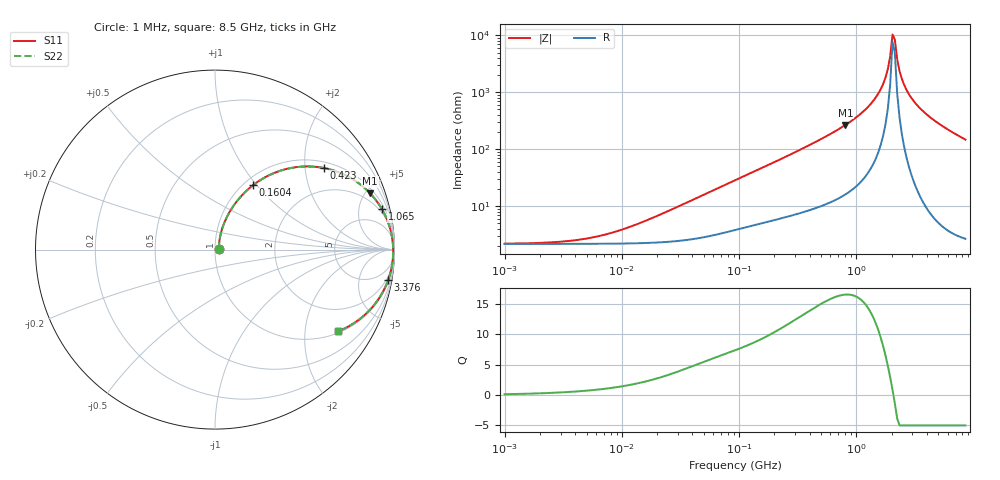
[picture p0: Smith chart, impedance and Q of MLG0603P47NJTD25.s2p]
! S-Parameter Data Generated by TDK Corporation
! Copyright(C) 2025 TDK Corporation.
! All Rights Reserved.
! TDK P/N: MLG0603P47NJTD25 (SMD / SMT Inductor (Coil))
! Property: L=47nH at 300MHz
! Size(LxWxT): 0.6x0.3x0.3mm
! Model Type: s2p (Touchstone File Format Version 1.0)
! Frequency: DC=Yes Start=1MHz Stop=8500MHz 198points Log-sweep
! Model Generated on Feb. 6, 2025
! Terms and conditions regarding TDK Simulation Models:
! 1)This simulation model is being provided solely for informational
!  purposes. Please refer to the specifications of the products in
!  terms of detailed characteristics of such products.
! 2)In no event shall TDK Corporation of any of its subsidiaries be
!  liable for any loss or damage arising, directly or indirectly,
!  from any information contained in this simulation model, including,
!  but not limited to loss or damages arising from any inaccuracies,
!  omissions or errors in connection with such information.
! 3)Any and all copyrights on this simulation model are owned by
!  TDK Corporation.  Duplication or redistribution of this simulation
!  model without prior written permission from TDK Corporation
!  is prohibited.
! 4)This simulation model is subject to any modification or change
!  without any prior notice.
! 5)Neither TDK Corporation nor any of its subsidiaries shall make any
!  warranty, express or implied, including but not limited to the
!  correctness, implied warranties of merchantability and fitness for
!  a particular purpose with respect to this simulation models.
! 6)The use of this simulation model shall be deemed to have consented
!  to the terms and conditions hereof.
! Port Assignments:
!  1 ---@@@--- 2
! Applicable Conditions:
!  Temperature = 25 degC
!  DC Bias Current = 0 A
!  Small Signal Operation
# Hz S MA R 50
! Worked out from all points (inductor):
!   197 points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, 1 MHz to 8.5 GHz, reference 50 ohm
!   read as one part in series: L = 50.5 nH near 22.04 MHz
!   highest Q = 16.6 at 807.2 MHz (marker M1), where L = 52.8 nH
!   self-resonance near 2.032 GHz
!   S11 on the Smith chart (normalised r, x): 1 MHz: 1.04, +0.01; 160.4 MHz: 1.10, +0.96; 423 MHz: 1.18, +2.52; 1.065 GHz: 1.51, +8.10; 3.376 GHz: 1, -11; 8.5 GHz: 1.05, -2.96
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1000000  0.02157 8.2  0.9787 -0.2  0.9787 -0.2  0.02157 8.2
4587603  0.02576 33.0  0.9785 -0.8  0.9785 -0.8  0.02576 33.0
9168677  0.03586 51.3  0.978 -1.6  0.978 -1.6  0.03586 51.3
2.10461e7  0.06914 67.1  0.9752 -3.7  0.9752 -3.7  0.06914 67.1
9.219544e7  0.2646 67.1  0.9295 -15.2  0.9295 -15.2  0.2646 67.1
1.604302e8  0.417 59.4  0.8658 -24.5  0.8658 -24.5  0.417 59.4
2.791662e8  0.6128 47.6  0.7411 -37.6  0.7411 -37.6  0.6128 47.6
4.229561e8  0.759 36.8  0.6 -49.2  0.6 -49.2  0.759 36.8
8.071757e8  0.919 20.0  0.3427 -66.5  0.3427 -66.5  0.919 20.0
1.064771e9  0.9571 13.6  0.236 -72.8  0.236 -72.8  0.9571 13.6
1.34121e9  0.9773 8.7  0.1516 -77.0  0.1516 -77.0  0.9773 8.7
1.613203e9  0.9872 4.9  0.08658 -79.0  0.08658 -79.0  0.9872 4.9
1.769233e9  0.9903 3.1  0.05471 -78.2  0.05471 -78.2  0.9903 3.1
1.940355e9  0.9922 1.3  0.02346 -70.0  0.02346 -70.0  0.9922 1.3
2.032026e9  0.9928 0.4  0.009566 -40.9  0.009566 -40.9  0.9928 0.4
2.128028e9  0.9931 -0.6  0.01184 53.8  0.01184 53.8  0.9931 -0.6
2.228565e9  0.993 -1.5  0.02644 74.0  0.02644 74.0  0.993 -1.5
2.444114e9  0.9922 -3.3  0.05805 80.6  0.05805 80.6  0.9922 -3.3
2.80715e9  0.9886 -6.1  0.1068 80.8  0.1068 80.8  0.9886 -6.1
3.37643e9  0.9794 -10.0  0.1741 78.2  0.1741 78.2  0.9794 -10.0
5.115526e9  0.9352 -19.7  0.3379 69.2  0.3379 69.2  0.9352 -19.7
8.5e9  0.8216 -33.7  0.5553 55.2  0.5553 55.2  0.8216 -33.7
